| IBIS file stm32g031_041_ufqfpn32.ibs
[IBIS ver]   4.2
[File name]  stm32g031_041_ufqfpn32.ibs
[File Rev]   1.2
[Date]   13-04-2022
[Source]   Data Created at STMicroelectronics
[Notes]   File originated from ELDO simulations.
[Disclaimer] This information is for modeling purpose only and is
   not guaranted. The information is subject to change without
   notice.
[Copyright] Copyright 2022 STMicroelectronics Inc.
|   Component stm32g031_041_ufqfpn32
[Component] stm32g031_041_ufqfpn32
[Manufacturer] STMicroelectronics
[Package]
| variable   typ   min   max
R_pkg   0.0   0.0   0.0
L_pkg   0.0H   0.0H   0.0H
C_pkg   0.0F   0.0F   0.0F
[Pin]   signal_name   model_name  R_pin L_pin C_pin
1 PB9 io6_i2c_ft
2 PC14-OSC32_IN io8prog2m25m50m120m_sudq_ft
3 PC15-OSC32_OUT io8prog2m25m50m120m_sudq_ft
4 VDD POWER
5 VSS GND
6 PF2-NRST io6reset
7 PA0 io6_ft
8 PA1 io6_ft
9 PA2 io6_ft
10 PA3 io6_ft
11 PA4 io6_ft
12 PA5 io6_ft
13 PA6 io6_ft
14 PA7 io6_ft
15 PB0 io6_ft
16 PB1 io6_ft
17 PB2 io6_ft
18 PA8 io6_ft
19 PA9 io6_i2c_ft
20 PC6 io6_ft
21 PA10 io6_i2c_ft
22 PA11 io6_i2c_ft
23 PA12 io6_i2c_ft
24 PA13 io6_ft
25 PA14-BOOT0 io6_ft
26 PA15 io6_ft
27 PB3 io6_ft
28 PB4 io6_ft
29 PB5 io6_ft
30 PB6 io6_i2c_ft
31 PB7 io6_i2c_ft
32 PB8 io6_i2c_ft
[Model Selector] io8prog2m25m50m120m_sudq_ft
iols8p_sudq_ft_pd_lv  "IO low speed, PD=40kOhm - 1P8V"
iols8p_sudq_ft_pu_lv  "IO low speed, PU=40kOhm - 1P8V"
iols8p_sudq_ft_lv  "IO low speed - 1P8V"
iols8p_sudq_ft_pd  "IO low speed, PD=40kOhm - 3P3V"
iols8p_sudq_ft_pu  "IO low speed, PU=40kOhm - 3P3V"
iols8p_sudq_ft  "IO low speed - 3P3V"
iofs8p_sudq_ft_pd_lv  "IO full speed, PD=40kOhm - 1P8V"
iofs8p_sudq_ft_pu_lv  "IO full speed, PU=40kOhm - 1P8V"
iofs8p_sudq_ft_lv  "IO full speed - 1P8V"
iofs8p_sudq_ft_pd  "IO full speed, PD=40kOhm - 3P3V"
iofs8p_sudq_ft_pu  "IO full speed, PU=40kOhm - 3P3V"
iofs8p_sudq_ft  "IO full speed - 3P3V"
ioms8p_sudq_ft_pd_lv  "IO medium speed, PD=40kOhm - 1P8V"
ioms8p_sudq_ft_pu_lv  "IO medium speed, PU=40kOhm - 1P8V"
ioms8p_sudq_ft_lv  "IO medium speed - 1P8V"
ioms8p_sudq_ft_pd  "IO medium speed, PD=40kOhm - 3P3V"
ioms8p_sudq_ft_pu  "IO medium speed, PU=40kOhm - 3P3V"
ioms8p_sudq_ft  "IO medium speed - 3P3V"
iohs8p_sudq_ft_pd_lv  "IO high speed, PD=40kOhm - 1P8V"
iohs8p_sudq_ft_pu_lv  "IO high speed, PU=40kOhm - 1P8V"
iohs8p_sudq_ft_lv  "IO high speed - 1P8V"
iohs8p_sudq_ft_pd  "IO high speed, PD=40kOhm - 3P3V"
iohs8p_sudq_ft_pu  "IO high speed, PU=40kOhm - 3P3V"
iohs8p_sudq_ft  "IO high speed - 3P3V"
[Model Selector] io6_ft
io6_ft_1v8_highspeed_pd  "GPIO-1.8V range - high speed - pull down"
io6_ft_1v8_fastspeed_pd  "GPIO-1.8V range - fast speed - pull down"
io6_ft_1v8_mediumspeed_pd  "GPIO-1.8V range - medium speed - pull down"
io6_ft_1v8_lowspeed_pd  "GPIO-1.8V range - low speed - pull down"
io6_ft_1v8_highspeed_pu  "GPIO-1.8V range - high speed - pull up"
io6_ft_1v8_fastspeed_pu  "GPIO-1.8V range - fast speed - pull up"
io6_ft_1v8_mediumspeed_pu  "GPIO-1.8V range - medium speed - pull up"
io6_ft_1v8_lowspeed_pu  "GPIO-1.8V range - low speed - pull up"
io6_ft_1v8_highspeed  "GPIO-1.8V range - high speed"
io6_ft_1v8_fastspeed  "GPIO-1.8V range - fast speed"
io6_ft_1v8_mediumspeed  "GPIO-1.8V range - medium speed"
io6_ft_1v8_lowspeed  "GPIO-1.8V range - low speed"
io6_ft_3v3_highspeed_pd  "GPIO-3.3V range - high speed - pull down"
io6_ft_3v3_fastspeed_pd  "GPIO-3.3V range - fast speed - pull down"
io6_ft_3v3_mediumspeed_pd  "GPIO-3.3V range - medium speed - pull down"
io6_ft_3v3_lowspeed_pd  "GPIO-3.3V range - low speed - pull down"
io6_ft_3v3_highspeed_pu  "GPIO-3.3V range - high speed - pull up"
io6_ft_3v3_fastspeed_pu  "GPIO-3.3V range - fast speed - pull up"
io6_ft_3v3_mediumspeed_pu  "GPIO-3.3V range - medium speed - pull up"
io6_ft_3v3_lowspeed_pu  "GPIO-3.3V range - low speed - pull up"
io6_ft_3v3_highspeed  "GPIO-3.3V range - high speed"
io6_ft_3v3_fastspeed  "GPIO-3.3V range - fast speed"
io6_ft_3v3_mediumspeed  "GPIO-3.3V range - medium speed"
io6_ft_3v3_lowspeed  "GPIO-3.3V range - low speed"
[Model Selector] io6_i2c_ft
io6_ft_1v8_highspeed_pd  "GPIO-1.8V range - high speed - pull down"
io6_ft_1v8_fastspeed_pd  "GPIO-1.8V range - fast speed - pull down"
io6_ft_1v8_mediumspeed_pd  "GPIO-1.8V range - medium speed - pull down"
io6_ft_1v8_lowspeed_pd  "GPIO-1.8V range - low speed - pull down"
io6_ft_1v8_highspeed_pu  "GPIO-1.8V range - high speed - pull up"
io6_ft_1v8_fastspeed_pu  "GPIO-1.8V range - fast speed - pull up"
io6_ft_1v8_mediumspeed_pu  "GPIO-1.8V range - medium speed - pull up"
io6_ft_1v8_lowspeed_pu  "GPIO-1.8V range - low speed - pull up"
io6_ft_1v8_highspeed  "GPIO-1.8V range - high speed"
io6_ft_1v8_fastspeed  "GPIO-1.8V range - fast speed"
io6_ft_1v8_mediumspeed  "GPIO-1.8V range - medium speed"
io6_ft_1v8_lowspeed  "GPIO-1.8V range - low speed"
io6_ft_3v3_highspeed_pd  "GPIO-3.3V range - high speed - pull down"
io6_ft_3v3_fastspeed_pd  "GPIO-3.3V range - fast speed - pull down"
io6_ft_3v3_mediumspeed_pd  "GPIO-3.3V range - medium speed - pull down"
io6_ft_3v3_lowspeed_pd  "GPIO-3.3V range - low speed - pull down"
io6_ft_3v3_highspeed_pu  "GPIO-3.3V range - high speed - pull up"
io6_ft_3v3_fastspeed_pu  "GPIO-3.3V range - fast speed - pull up"
io6_ft_3v3_mediumspeed_pu  "GPIO-3.3V range - medium speed - pull up"
io6_ft_3v3_lowspeed_pu  "GPIO-3.3V range - low speed - pull up"
io6_ft_3v3_highspeed  "GPIO-3.3V range - high speed"
io6_ft_3v3_fastspeed  "GPIO-3.3V range - fast speed"
io6_ft_3v3_mediumspeed  "GPIO-3.3V range - medium speed"
io6_ft_3v3_lowspeed  "GPIO-3.3V range - low speed"
io6_ft_1v8_highi2c_pd   "GPIO-1.8V range - high   speed i2c mode - pd"
io6_ft_1v8_fasti2c_pd   "GPIO-1.8V range - fast   speed i2c mode - pd"
io6_ft_1v8_mediumi2c_pd  "GPIO-1.8V range - medium speed i2c mode - pd"
io6_ft_1v8_lowi2c_pd   "GPIO-1.8V range - low   speed i2c mode - pd"
io6_ft_1v8_highi2c_pu   "GPIO-1.8V range - high   speed i2c mode - pu"
io6_ft_1v8_fasti2c_pu   "GPIO-1.8V range - fast   speed i2c mode - pu"
io6_ft_1v8_mediumi2c_pu  "GPIO-1.8V range - medium speed i2c mode - pu"
io6_ft_1v8_lowi2c_pu   "GPIO-1.8V range - low   speed i2c mode - pu"
io6_ft_1v8_highi2c   "GPIO-1.8V range - high   speed i2c mode"
io6_ft_1v8_fasti2c   "GPIO-1.8V range - fast   speed i2c mode"
io6_ft_1v8_mediumi2c   "GPIO-1.8V range - medium speed i2c mode"
io6_ft_1v8_lowi2c   "GPIO-1.8V range - low   speed i2c mode"
io6_ft_3v3_highi2c_pd   "GPIO-3.3V range - high   speed i2c mode - pd"
io6_ft_3v3_fasti2c_pd   "GPIO-3.3V range - fast   speed i2c mode - pd"
io6_ft_3v3_mediumi2c_pd  "GPIO-3.3V range - medium speed i2c mode - pd"
io6_ft_3v3_lowi2c_pd   "GPIO-3.3V range - low   speed i2c mode - pd"
io6_ft_3v3_highi2c_pu   "GPIO-3.3V range - high   speed i2c mode - pu"
io6_ft_3v3_fasti2c_pu   "GPIO-3.3V range - fast   speed i2c mode - pu"
io6_ft_3v3_mediumi2c_pu  "GPIO-3.3V range - medium speed i2c mode - pu"
io6_ft_3v3_lowi2c_pu   "GPIO-3.3V range - low   speed i2c mode - pu"
io6_ft_3v3_highi2c   "GPIO-3.3V range - high   speed i2c mode"
io6_ft_3v3_fasti2c   "GPIO-3.3V range - fast   speed i2c mode"
io6_ft_3v3_mediumi2c   "GPIO-3.3V range - medium speed i2c mode"
io6_ft_3v3_lowi2c   "GPIO-3.3V range - low   speed i2c mode"
io6_i2c_ft_1v8_pd  "GPIO-1.8V I2C fm+ - pd"
io6_i2c_ft_3v3_pd  "GPIO-3.3V I2C fm+ - pd"
io6_i2c_ft_1v8_pu  "GPIO-1.8V I2C fm+ - pu"
io6_i2c_ft_3v3_pu  "GPIO-3.3V I2C fm+ - pu"
io6_i2c_ft_1v8   "GPIO-1.8V I2C fm+"
io6_i2c_ft_3v3   "GPIO-3.3V I2C fm+"
[Model Selector] io6reset
io6_ft_1v8_highspeed_pd  "GPIO-1.8V range - high speed - pull down"
io6_ft_1v8_fastspeed_pd  "GPIO-1.8V range - fast speed - pull down"
io6_ft_1v8_mediumspeed_pd  "GPIO-1.8V range - medium speed - pull down"
io6_ft_1v8_lowspeed_pd  "GPIO-1.8V range - low speed - pull down"
io6_ft_1v8_highspeed_pu  "GPIO-1.8V range - high speed - pull up"
io6_ft_1v8_fastspeed_pu  "GPIO-1.8V range - fast speed - pull up"
io6_ft_1v8_mediumspeed_pu  "GPIO-1.8V range - medium speed - pull up"
io6_ft_1v8_lowspeed_pu  "GPIO-1.8V range - low speed - pull up"
io6_ft_1v8_highspeed  "GPIO-1.8V range - high speed"
io6_ft_1v8_fastspeed  "GPIO-1.8V range - fast speed"
io6_ft_1v8_mediumspeed  "GPIO-1.8V range - medium speed"
io6_ft_1v8_lowspeed  "GPIO-1.8V range - low speed"
io6_ft_3v3_highspeed_pd  "GPIO-3.3V range - high speed - pull down"
io6_ft_3v3_fastspeed_pd  "GPIO-3.3V range - fast speed - pull down"
io6_ft_3v3_mediumspeed_pd  "GPIO-3.3V range - medium speed - pull down"
io6_ft_3v3_lowspeed_pd  "GPIO-3.3V range - low speed - pull down"
io6_ft_3v3_highspeed_pu  "GPIO-3.3V range - high speed - pull up"
io6_ft_3v3_fastspeed_pu  "GPIO-3.3V range - fast speed - pull up"
io6_ft_3v3_mediumspeed_pu  "GPIO-3.3V range - medium speed - pull up"
io6_ft_3v3_lowspeed_pu  "GPIO-3.3V range - low speed - pull up"
io6_ft_3v3_highspeed  "GPIO-3.3V range - high speed"
io6_ft_3v3_fastspeed  "GPIO-3.3V range - fast speed"
io6_ft_3v3_mediumspeed  "GPIO-3.3V range - medium speed"
io6_ft_3v3_lowspeed  "GPIO-3.3V range - low speed"
ioreset_1v2_pu  "RESET 1.2V range with PU"
ioreset_1v2  "RESET 1.2V range"
ioreset_1v8_pu  "RESET 1.8V range with PU"
ioreset_1v8  "RESET 1.8V range"
ioreset_3v3_pu  "RESET 3.3V range with PU"
ioreset_3v3  "RESET 3.3V range"
[Define Package Model]  466-ufqfpn-5x5-32-220413
[Manufacturer]  Unknown
[OEM]  Unknown
[Description]  None
[Number Of Pins]  32
[Pin Numbers]
| Pin Num   Terminal Name
7 | PA0
8 | PA1
9 | PA2
10 | PA3
11 | PA4
12 | PA5
13 | PA6
14 | PA7
18 | PA8
19 | PA9
21 | PA10
22 | PA11
23 | PA12
24 | PA13
25 | PA14
26 | PA15
15 | PB0
16 | PB1
17 | PB2
27 | PB3
28 | PB4
29 | PB5
30 | PB6
31 | PB7
32 | PB8
1 | PB9
20 | PC6
2 | PC14
3 | PC15
6 | PF2_NRST
4 | VDD
5 | VSS
[Model Data]
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[End Model Data]
[End Package Model]
| Models and submodels in the file (84): iols8p_sudq_ft_pd_lv (I/O), iols8p_sudq_ft_pu_lv (I/O), iols8p_sudq_ft_lv (I/O), iols8p_sudq_ft_pd (I/O), iols8p_sudq_ft_pu (I/O), iols8p_sudq_ft (I/O), iofs8p_sudq_ft_pd_lv (I/O), iofs8p_sudq_ft_pu_lv (I/O), iofs8p_sudq_ft_lv (I/O), iofs8p_sudq_ft_pd (I/O), iofs8p_sudq_ft_pu (I/O), iofs8p_sudq_ft (I/O), ioms8p_sudq_ft_pd_lv (I/O), ioms8p_sudq_ft_pu_lv (I/O), ioms8p_sudq_ft_lv (I/O), ioms8p_sudq_ft_pd (I/O), ioms8p_sudq_ft_pu (I/O), ioms8p_sudq_ft (I/O), iohs8p_sudq_ft_pd_lv (I/O), iohs8p_sudq_ft_pu_lv (I/O), iohs8p_sudq_ft_lv (I/O), iohs8p_sudq_ft_pd (I/O), iohs8p_sudq_ft_pu (I/O), iohs8p_sudq_ft (I/O), io6_ft_1v8_highspeed_pd (I/O), io6_ft_1v8_fastspeed_pd (I/O), io6_ft_1v8_mediumspeed_pd (I/O), io6_ft_1v8_lowspeed_pd (I/O), io6_ft_1v8_highspeed_pu (I/O), io6_ft_1v8_fastspeed_pu (I/O), io6_ft_1v8_mediumspeed_pu (I/O), io6_ft_1v8_lowspeed_pu (I/O), io6_ft_1v8_highspeed (I/O), io6_ft_1v8_fastspeed (I/O), io6_ft_1v8_mediumspeed (I/O), io6_ft_1v8_lowspeed (I/O), io6_ft_3v3_highspeed_pd (I/O), io6_ft_3v3_fastspeed_pd (I/O), io6_ft_3v3_mediumspeed_pd (I/O), io6_ft_3v3_lowspeed_pd (I/O), io6_ft_3v3_highspeed_pu (I/O), io6_ft_3v3_fastspeed_pu (I/O), io6_ft_3v3_mediumspeed_pu (I/O), io6_ft_3v3_lowspeed_pu (I/O), io6_ft_3v3_highspeed (I/O), io6_ft_3v3_fastspeed (I/O), io6_ft_3v3_mediumspeed (I/O), io6_ft_3v3_lowspeed (I/O), io6_i2c_ft_1v8_pd (I/O_open_drain), io6_i2c_ft_3v3_pd (I/O_open_drain), io6_i2c_ft_1v8_pu (I/O_open_drain), io6_i2c_ft_3v3_pu (I/O_open_drain), io6_i2c_ft_1v8 (I/O_open_drain), io6_i2c_ft_3v3 (I/O_open_drain), io6_ft_1v8_highi2c_pd (I/O_open_drain), io6_ft_1v8_fasti2c_pd (I/O_open_drain), io6_ft_1v8_mediumi2c_pd (I/O_open_drain), io6_ft_1v8_lowi2c_pd (I/O_open_drain), io6_ft_1v8_highi2c_pu (I/O_open_drain), io6_ft_1v8_fasti2c_pu (I/O_open_drain), io6_ft_1v8_mediumi2c_pu (I/O_open_drain), io6_ft_1v8_lowi2c_pu (I/O_open_drain), io6_ft_1v8_highi2c (I/O_open_drain), io6_ft_1v8_fasti2c (I/O_open_drain), io6_ft_1v8_mediumi2c (I/O_open_drain), io6_ft_1v8_lowi2c (I/O_open_drain), io6_ft_3v3_highi2c_pd (I/O_open_drain), io6_ft_3v3_fasti2c_pd (I/O_open_drain), io6_ft_3v3_mediumi2c_pd (I/O_open_drain), io6_ft_3v3_lowi2c_pd (I/O_open_drain), io6_ft_3v3_highi2c_pu (I/O_open_drain), io6_ft_3v3_fasti2c_pu (I/O_open_drain), io6_ft_3v3_mediumi2c_pu (I/O_open_drain), io6_ft_3v3_lowi2c_pu (I/O_open_drain), io6_ft_3v3_highi2c (I/O_open_drain), io6_ft_3v3_fasti2c (I/O_open_drain), io6_ft_3v3_mediumi2c (I/O_open_drain), io6_ft_3v3_lowi2c (I/O_open_drain), ioreset_1v2_pu (I/O_open_drain), ioreset_1v2 (I/O_open_drain)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
